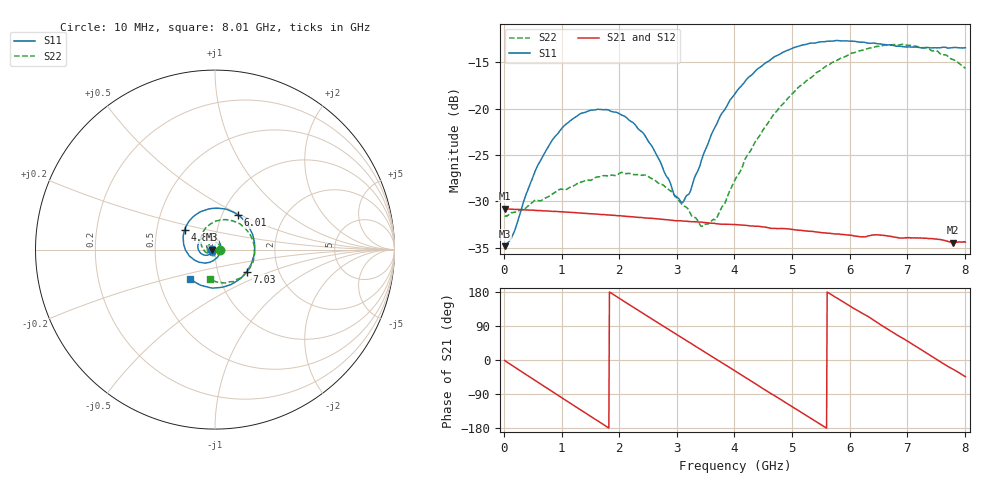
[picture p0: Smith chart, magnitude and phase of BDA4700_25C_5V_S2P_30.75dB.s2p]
!Agilent Technologies,E5071B,MY42404982,A.09.10
!Date: Mon Oct 20 13:42:06 2025
!Data & Calibration Information:
!Freq	S11:SOLT2(ON)	S21:SOLT2(ON)	S12:SOLT2(ON)	S22:SOLT2(ON)
# Hz S RI R 50
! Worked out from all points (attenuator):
!   801 points, 10 MHz to 8.01 GHz, reference 50 ohm
!   highest |S21| = -30.81 dB at 10 MHz (marker M1); lowest = -34.5 dB at 7.8 GHz (marker M2)
!   lowest |S11| = -34.9 dB at 10 MHz (marker M3), VSWR 1.04, Z = 48.2 - j0.0942 ohm
!   |S11| at or under -10 dB: start of sweep to end of sweep
!   |S22| runs from -32.7 to -13.1 dB; largest |S21 - S12| = 0.00024
!   S11 on the Smith chart (normalised r, x): 10 MHz: 0.96, -0.00; 4.85 GHz: 0.70, +0.16; 6.01 GHz: 1.19, +0.48; 7.03 GHz: 1.37, -0.36; 8.01 GHz: 0.72, -0.25
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1e7  -0.0181 -0.000976  0.0288 -0.000626  0.0288 -0.000635  0.0263 -0.000836
1.6e8  -0.0188 -0.00945  0.0275 -0.008  0.0275 -0.008  0.0265 -0.00755
5.3e8  -0.035 -0.0285  0.017 -0.0226  0.017 -0.0226  0.0162 -0.0275
7.7e8  -0.0539 -0.0316  0.00641 -0.0272  0.00645 -0.0273  0.00112 -0.0335
1.35e9  -0.0945 0.00481  -0.0188 -0.0198  -0.0189 -0.0197  -0.036 -0.0179
2.09e9  -0.0518 0.0748  -0.0237 0.0114  -0.0237 0.0114  -0.0293 0.0338
2.42e9  -0.00886 0.0731  -0.0138 0.0217  -0.0138 0.0218  -0.00515 0.0433
2.68e9  0.0189 0.0505  -0.00331 0.0251  -0.00327 0.0251  0.0125 0.0375
2.96e9  0.0316 0.0125  0.00818 0.0235  0.00819 0.0235  0.0253 0.0228
3.11e9  0.0296 -0.0103  0.0136 0.0206  0.0136 0.0206  0.028 0.0109
3.41e9  0.00464 -0.05  0.0215 0.0115  0.0216 0.0115  0.0205 -0.0113
3.54e9  -0.0131 -0.0631  0.0233 0.00653  0.0233 0.00647  0.0131 -0.02
3.7e9  -0.0415 -0.0725  0.0239 0.000215  0.0239 0.000103  -0.000414 -0.0259
4.01e9  -0.1015 -0.0645  0.0207 -0.0114  0.0207 -0.0114  -0.032 -0.0257
4.85e9  -0.1694 0.1101  -0.0072 -0.0213  -0.0071 -0.0214  -0.0757 0.075
5.35e9  -0.0739 0.2137  -0.0199 -0.00874  -0.0199 -0.00881  -0.0156 0.1476
6.01e9  0.1287 0.1919  -0.0163 0.0128  -0.0164 0.0128  0.1331 0.1463
6.68e9  0.221 -0.00895  0.00375 0.0202  0.00384 0.0202  0.2197 0.000483
7.03e9  0.1762 -0.1236  0.0136 0.0148  0.0137 0.0147  0.1989 -0.0931
7.44e9  0.0562 -0.2054  0.0197 0.00286  0.0197 0.00286  0.1164 -0.1683
7.8e9  -0.0734 -0.2009  0.0171 -0.00793  0.0172 -0.00802  0.0209 -0.1826
8.01e9  -0.137 -0.1634  0.0136 -0.0132  0.0137 -0.0133  -0.0299 -0.1623
